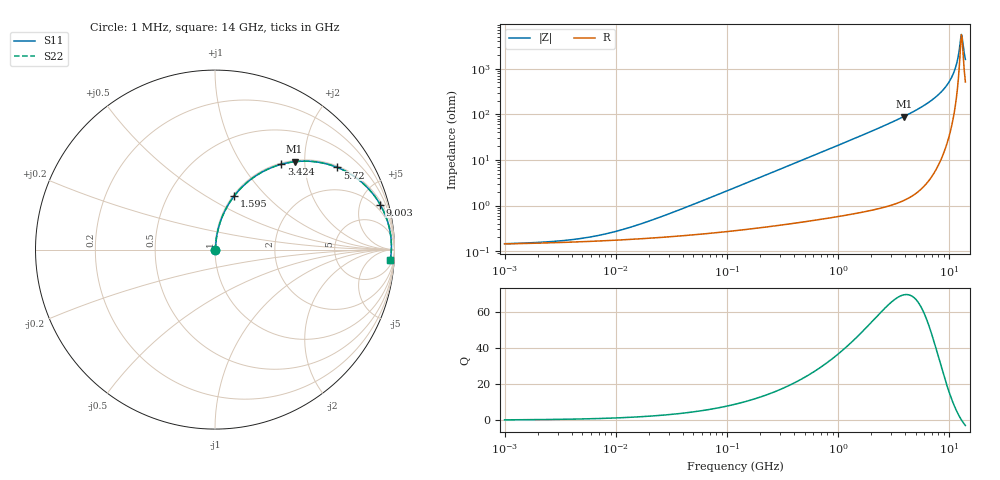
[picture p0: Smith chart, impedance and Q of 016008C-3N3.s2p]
# MHz S MA R 50
!Freq  MagS11  AngS11  MagS21  AngS21  MagS12  AngS12  MagS22  AngS22
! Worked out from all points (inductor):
!   801 points, 1 MHz to 14 GHz, reference 50 ohm
!   read as one part in series: L = 3.3 nH near 30 MHz
!   highest Q = 69.2 at 3.905 GHz (marker M1), where L = 3.63 nH
!   self-resonance near 12.88 GHz
!   S11 on the Smith chart (normalised r, x): 1 MHz: 1.00, +0.00; 1.595 GHz: 1.01, +0.67; 3.424 GHz: 1.02, +1.53; 5.72 GHz: 1.05, +2.95; 9.003 GHz: 1.30, +7.24; 14 GHz: 11, -30
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1  0.001451 8.2  0.9986 -0.0  0.9986 -0.0  0.001451 8.2
2.506483  0.001603 18.9  0.9985 -0.0  0.9985 -0.0  0.001603 18.9
4.948533  0.001904 32.5  0.9984 -0.1  0.9984 -0.1  0.001904 32.5
10.37054  0.002764 50.8  0.9983 -0.1  0.9983 -0.1  0.002764 50.8
24.19749  0.005383 68.2  0.998 -0.3  0.998 -0.3  0.005383 68.2
119.742  0.02491 82.1  0.9969 -1.4  0.9969 -1.4  0.02491 82.1
585.5183  0.1203 80.9  0.9881 -6.9  0.9881 -6.9  0.1203 80.9
1038.265  0.2107 76.3  0.9719 -12.2  0.9719 -12.2  0.2107 76.3
1595.453  0.3165 70.4  0.942 -18.4  0.942 -18.4  0.3165 70.4
2863.085  0.5259 57.4  0.8423 -31.7  0.8423 -31.7  0.5259 57.4
3424.318  0.6027 52.1  0.7891 -37.1  0.7891 -37.1  0.6027 52.1
3904.662  0.6606 47.8  0.7413 -41.3  0.7413 -41.3  0.6606 47.8
5720.428  0.8216 33.8  0.5569 -55.2  0.5569 -55.2  0.8216 33.8
7349.612  0.9062 23.7  0.4023 -64.9  0.4023 -64.9  0.9062 23.7
9002.634  0.954 15.2  0.2632 -72.4  0.2632 -72.4  0.954 15.2
10143.7  0.9718 10.2  0.1778 -75.8  0.1778 -75.8  0.9718 10.2
11027.44  0.9794 6.7  0.1174 -76.6  0.1174 -76.6  0.9794 6.7
11705.45  0.9824 4.2  0.07437 -74.2  0.07437 -74.2  0.9824 4.2
12425.14  0.9832 1.7  0.03336 -59.0  0.03336 -59.0  0.9832 1.7
12725.26  0.983 0.7  0.02053 -33.8  0.02053 -33.8  0.983 0.7
13189.09  0.982 -0.8  0.02309 38.4  0.02309 38.4  0.982 -0.8
14000  0.9787 -3.3  0.06131 68.0  0.06131 68.0  0.9787 -3.3
